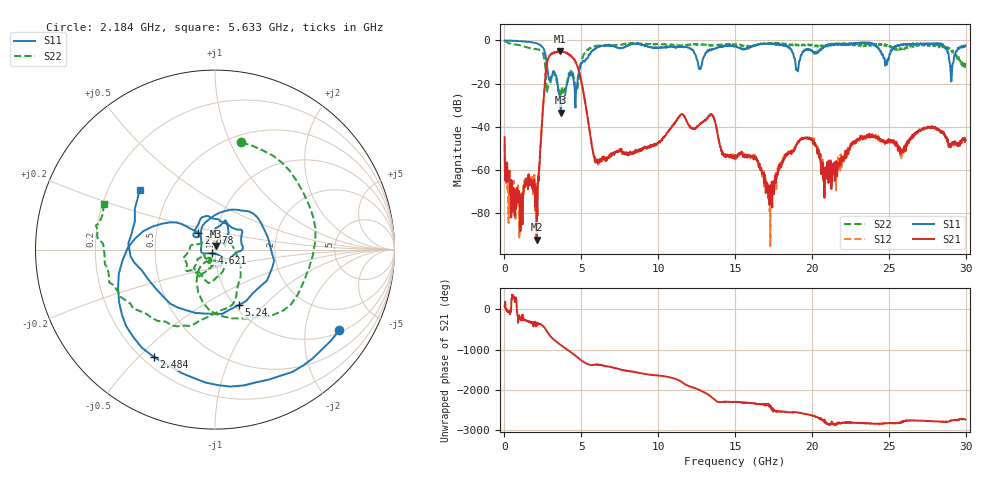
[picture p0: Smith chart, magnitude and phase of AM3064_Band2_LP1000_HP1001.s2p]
# Hz S DB R 50.0
!freq dBS11 angS11 dBS21 angS21 dBS12 angS12 dBS22 angS22
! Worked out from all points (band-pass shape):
!   1600 points, 10 MHz to 29.98 GHz, reference 50 ohm
!   highest |S21| = -5.02 dB at 3.59 GHz (marker M1); lowest = -92.1 dB at 2.091 GHz (marker M2)
!   |S21| within 3 dB of the highest: 2.864 GHz to 4.433 GHz (1.569 GHz wide, 43 % of centre)
!   lowest |S11| = -33.4 dB at 3.665 GHz (marker M3), VSWR 1.04, Z = 50.7 + j2.04 ohm
!   |S11| at or under -10 dB: 2.735 GHz to 5.084 GHz (2.349 GHz wide, 60.1 % of centre); 12.57 GHz to 12.86 GHz (291.1 MHz wide, 2.29 % of centre); 28.95 GHz to 29.21 GHz (257.4 MHz wide, 0.885 % of centre)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
!   |S22| runs from -25.5 to -0.3 dB; largest |S21 - S12| = 0.016
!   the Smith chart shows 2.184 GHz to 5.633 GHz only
!   S11 on the Smith chart (normalised r, x): 2.184 GHz: 1.08, -3.03; 2.484 GHz: 0.24, -0.55; 2.878 GHz: 0.82, +0.16; 4.621 GHz: 0.96, -0.04; 5.24 GHz: 1.04, -0.73; 5.633 GHz: 0.33, +0.31
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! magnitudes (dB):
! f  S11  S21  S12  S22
! 10 MHz  0.0  -44.8  -48.3  -0.3
! 647.3 MHz  -0.3  -68.7  -81.7  -1.8
! 2.091 GHz  -1.3  -92.1  -66.5  -4.2
! 2.184 GHz  -1.7  -64.0  -65.2  -4.2
! 2.484 GHz  -3.2  -33.5  -33.5  -5.6
! 2.878 GHz  -17.5  -7.8  -7.7  -20.8
! 3.59 GHz  -26.0  -5.0  -5.1  -23.4
! 3.665 GHz  -33.4  -5.3  -5.2  -24.7
! 4.621 GHz  -31.2  -9.8  -9.9  -22.9
! 5.015 GHz  -10.6  -19.4  -19.5  -9.6
! 5.24 GHz  -9.5  -28.2  -28.2  -5.7
! 5.633 GHz  -5.4  -45.9  -46.1  -3.5
! 6.083 GHz  -3.0  -55.9  -56.1  -2.5
! 10 GHz  -3.4  -47.3  -47.5  -1.8
! 13.43 GHz  -4.5  -34.3  -34.1  -2.3
! 15 GHz  -2.5  -54.7  -53.5  -1.9
! 16.34 GHz  -2.3  -55.0  -54.3  -2.3
! 17.31 GHz  -1.6  -73.0  -69.6  -1.5
! 19.99 GHz  -4.6  -45.3  -46.1  -2.0
! 20.89 GHz  -2.3  -62.9  -58.9  -2.8
! 25 GHz  -8.4  -45.8  -47.1  -2.2
! 29.98 GHz  -2.3  -46.0  -45.8  -10.5
